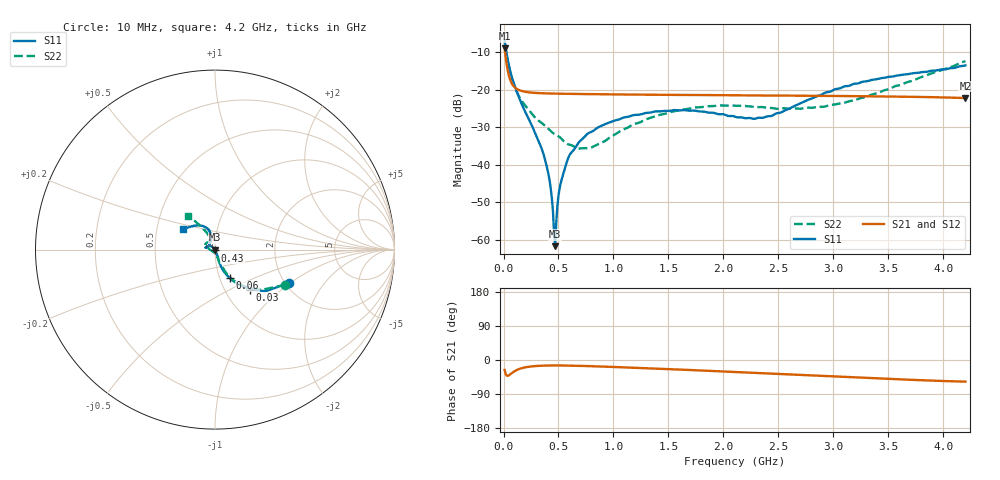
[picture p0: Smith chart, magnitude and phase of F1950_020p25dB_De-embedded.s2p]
! Integrated Device Technology
! Corporate Headquarters
! 6024 Silver Creek Valley Road
! San Jose, CA 95138  USA
! Phone:  1-408-284-8200
! Toll Free:  1-800-223-1366
! Webpage:  http://www.idt.com/
! Timing and RF Division
! 515 Groton Road, Suite 102
! Westford, MA 01886-6024
! Device:  F1950
! Description: 7-bit 0.25 dB Digital Step Attenuator
! Frequency:  150.0 -  4000.00 MHz
! Package:  4x4 mm Thin QFN Plastic Package: 24 pin
! Ports:  2 RF, 12 DC
!  Pin  1  = D0
!  Pin  2  = VDD
!  Pin  3  = Vmode
!  Pin  4  = GND
!  Pin  5  = RF1  =  Port 1
!  Pin  6  = GND
!  Pin  7  = GND
!  Pin  8  = GND
!  Pin  9  = GND
!  Pin 10  = GND
!  Pin 11  = GND
!  Pin 12  = GND
!  Pin 13  = GND
!  Pin 14  = RF2  =  Port 2
!  Pin 15  = GND
!  Pin 16  = LE
!  Pin 17  = CLK
!  Pin 18  = DATE
!  Pin 19  = D6
!  Pin 20  = D5
!  Pin 21  = D4
!  Pin 22  = D3
!  Pin 23  = D2
!  Pin 24  = D1
! State:  81
! Atten State:  20.25 dB
! Voltage:  +5.00 Volts
! Current:  Not Measured mA
! Data:  The device was measured on a the F195X evaluation board which has
!  individual transmission lines to the RF pins.  Data was collected
!  using a calibrated network analyzer.  The evaluation board was
!  de-embedded using a TRL calibration technique.
!  The reference plane is the edge of the package pin.
! Misc:  Board 2019
!  Action Tracker AT0250
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# GHz S dB R 50
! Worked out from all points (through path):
!   420 points, 10 MHz to 4.2 GHz, reference 50 ohm
!   highest |S21| = -8.97 dB at 10 MHz (marker M1); lowest = -22.2 dB at 4.2 GHz (marker M2)
!   group delay of S21, straight-line fit = 29.2 ps
!   lowest |S11| = -61.7 dB at 470 MHz (marker M3), VSWR 1.00, Z = 49.9 - j0.00961 ohm
!   |S11| at or under -10 dB: 26.92 MHz to end of sweep
!   |S22| runs from -35.7 to -7.2 dB; largest |S21 - S12| = 0.00015
!   S11 on the Smith chart (normalised r, x): 10 MHz: 2.10, -0.98; 30 MHz: 1.31, -0.64; 60 MHz: 1.12, -0.37; 430 MHz: 1.00, -0.01; 4.2 GHz: 0.68, +0.17
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0.01  -6.86 -24.1  -8.97 -26.2  -8.97 -26.2  -7.18 -26.7
0.03  -10.56 -48.6  -13.46 -41.2  -13.46 -41.2  -11.09 -49.4
0.06  -14.93 -62.5  -17.29 -38.2  -17.29 -38.2  -15.17 -61.9
0.15  -22.73 -71.2  -20.20 -23.0  -20.20 -23.0  -22.26 -70.1
0.35  -35.98 -66.4  -20.95 -15.0  -20.94 -15.0  -28.93 -77.0
0.4  -41.33 -67.4  -21.00 -14.6  -21.00 -14.6  -30.20 -77.8
0.43  -46.48 -72.7  -21.02 -14.5  -21.02 -14.5  -31.03 -80.0
0.45  -52.56 -81.2  -21.04 -14.4  -21.03 -14.4  -31.55 -82.6
0.47  -61.74 -173.2  -21.05 -14.4  -21.05 -14.4  -31.92 -85.4
0.48  -55.25 147.8  -21.05 -14.4  -21.05 -14.4  -32.09 -86.5
0.51  -46.33 136.5  -21.07 -14.5  -21.07 -14.5  -32.63 -88.6
0.56  -40.81 132.8  -21.09 -14.6  -21.09 -14.6  -34.10 -94.2
0.61  -37.01 134.8  -21.12 -14.9  -21.12 -14.9  -34.73 -104.5
0.71  -33.32 136.8  -21.15 -15.6  -21.15 -15.6  -35.63 -123.8
0.99  -28.45 147.2  -21.25 -18.2  -21.25 -18.3  -32.35 -173.0
1.41  -25.79 163.6  -21.35 -23.0  -21.35 -23.0  -26.79 164.1
1.73  -25.56 169.3  -21.42 -26.8  -21.41 -26.9  -24.81 155.3
2.11  -27.25 159.1  -21.49 -31.9  -21.49 -31.9  -24.29 145.6
2.43  -27.04 126.9  -21.55 -35.8  -21.55 -35.9  -24.86 135.3
2.81  -22.26 105.4  -21.63 -41.0  -21.62 -41.0  -24.81 120.0
3.51  -16.55 117.7  -21.81 -50.0  -21.81 -50.1  -19.79 115.9
4.2  -13.50 146.3  -22.22 -57.0  -22.22 -57.1  -12.36 128.2
